(* Logix 5000 AddOnInstructionDefinition export AKD_Set_Mode; software revision 19.01 *)

TYPE AKD_Status :
STRUCT
   Profile_In_Progress : BOOL;
   Block_In_Execution : BOOL;
   On_Target_Position : BOOL;
   General_Fault : BOOL;
   Current_Direction : BOOL;
   Home_Level : BOOL;
   Reg_Level : BOOL;
   Enable : BOOL;
   Fault_Input_Fault : BOOL;
   Fwd_Limit : BOOL;
   Rev_Limit : BOOL;
   Positive_Limit : BOOL;
   Negative_Limit : BOOL;
   FE_Fault : BOOL;
   Block_Fault : BOOL;
   Load_Complete : BOOL;
END_STRUCT
END_TYPE

TYPE AKD_Control :
STRUCT
   Load_Data_Start_Profile : BOOL;
   Start_Block : BOOL;
   Incremental : BOOL;
   Direction : BOOL;
   Smooth_Stop : BOOL;
   Hard_Stop : BOOL;
   Reg_Arm : BOOL;
   Enable : BOOL;
END_STRUCT
END_TYPE

TYPE AKD_Axis :
STRUCT
   Control : AKD_Control;
   Status : AKD_Status;
   Input : AB:ETHERNET_MODULE_SINT_64Bytes:I:0;
   Output : AB:ETHERNET_MODULE_SINT_64Bytes:O:0;
   ResponseMsgType : SINT;
   CommandTimeout : INT;
   PositionFeedback : DINT;
   VelocityFeedback : DINT;
END_STRUCT
END_TYPE

ADD_ON_INSTRUCTION AKD_Get_Attribute   (* revision 2.1, ExecutePrescan, ExecuteEnableInFalse *)
VAR_OUTPUT
   DN : BOOL; {access Read Only, visible}
   ER : BOOL; {access Read Only, visible}
END_VAR
VAR_IN_OUT
   Axis : AKD_Axis; {required}
END_VAR
VAR_INPUT
   Attribute_Number : INT; {visible}
END_VAR
VAR_OUTPUT
   Attribute_Value : DINT; {access Read Only, required}
END_VAR
VAR
   Command_Timeout : TIMER := (PRE := 100);
   OS_LoadStart : BOOL;
   ErrorSource : SINT;
END_VAR

ROUTINE EnableInFalse   (* ladder *)
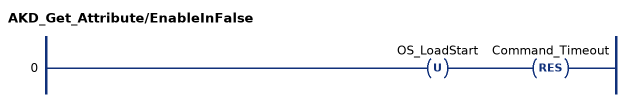
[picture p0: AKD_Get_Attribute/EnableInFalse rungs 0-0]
   0: OTU(OS_LoadStart)RES(Command_Timeout);
END_ROUTINE

ROUTINE Logic   (* ladder *)
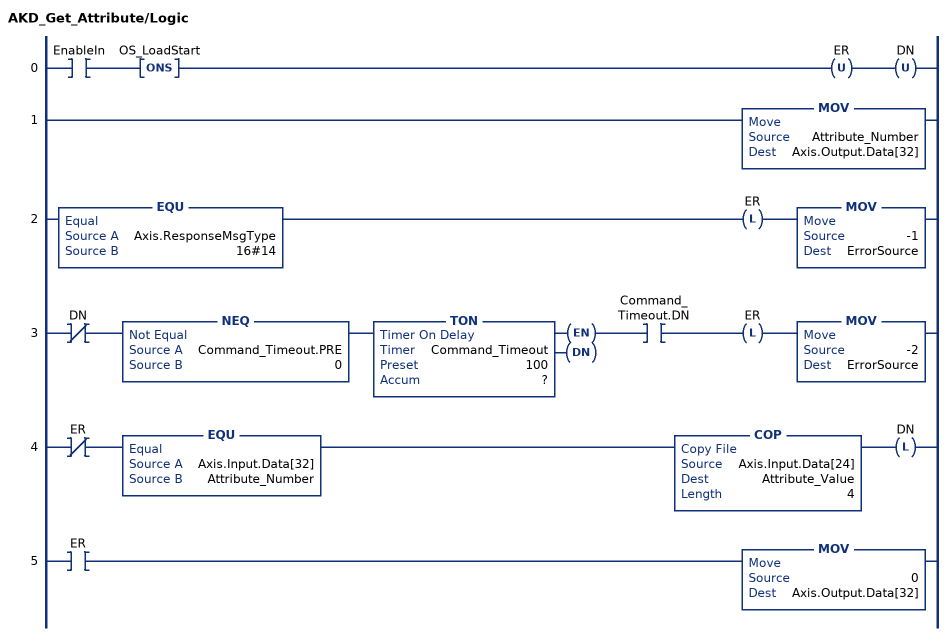
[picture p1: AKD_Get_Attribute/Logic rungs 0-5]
   0: XIC(EnableIn)ONS(OS_LoadStart)OTU(ER)OTU(DN);
   1: MOV(Attribute_Number,Axis.Output.Data[32]);
   2: EQU(Axis.ResponseMsgType,16#14)OTL(ER)MOV(-1,ErrorSource);
   3: XIO(DN)NEQ(Command_Timeout.PRE,0)TON(Command_Timeout,?,?)XIC(Command_Timeout.DN)OTL(ER)MOV(-2,ErrorSource);
   4: XIO(ER)EQU(Axis.Input.Data[32],Attribute_Number)COP(Axis.Input.Data[24],Attribute_Value,4)OTL(DN);
   5: XIC(ER)MOV(0,Axis.Output.Data[32]);
END_ROUTINE

ROUTINE Prescan   (* ladder *)
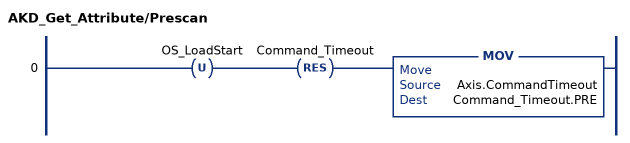
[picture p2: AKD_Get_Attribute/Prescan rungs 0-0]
   0: OTU(OS_LoadStart)RES(Command_Timeout)MOV(Axis.CommandTimeout,Command_Timeout.PRE);
END_ROUTINE
END_ADD_ON_INSTRUCTION

ADD_ON_INSTRUCTION AKD_Set_Attribute   (* revision 2.1, ExecutePrescan, ExecuteEnableInFalse *)
VAR_OUTPUT
   DN : BOOL; {access Read Only, visible}
   ER : BOOL; {access Read Only, visible}
END_VAR
VAR_IN_OUT
   Axis : AKD_Axis; {required}
END_VAR
VAR_INPUT
   Attribute_Number : INT; {visible}
   Attribute_Value : DINT; {required}
END_VAR
VAR
   Command_Timeout : TIMER := (PRE := 200);
   Command_Message_Type : SINT;
   Command_Axis_Number : SINT;
   Step : SINT;
   Command_Bytes : SINT[8];
   OS_LoadStart : BOOL;
END_VAR

ROUTINE EnableInFalse   (* ladder *)
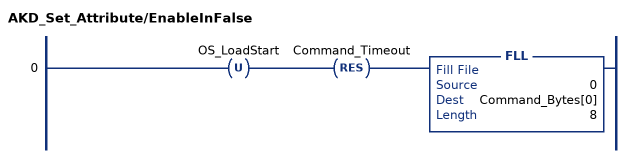
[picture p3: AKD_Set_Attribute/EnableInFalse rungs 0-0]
   0: OTU(OS_LoadStart)RES(Command_Timeout)FLL(0,Command_Bytes[0],8);
END_ROUTINE

ROUTINE Logic   (* ladder *)
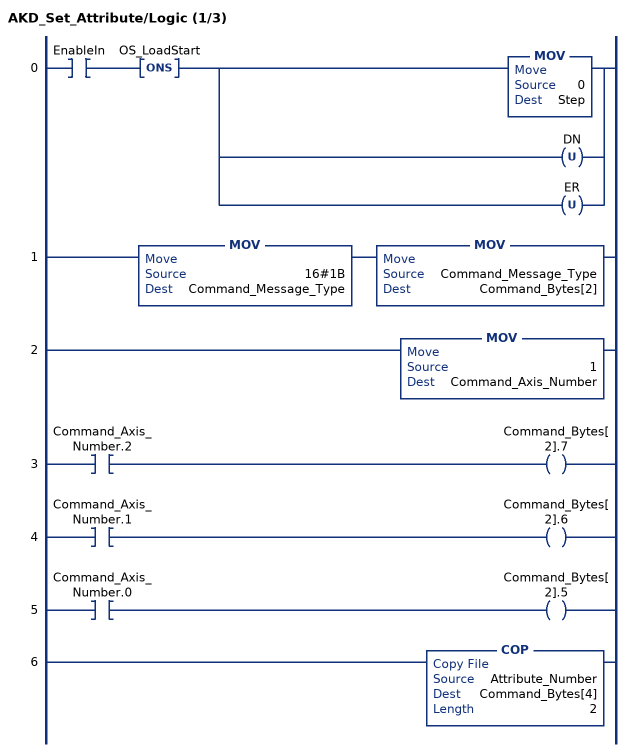
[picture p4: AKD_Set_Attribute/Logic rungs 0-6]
   0: XIC(EnableIn)ONS(OS_LoadStart)[MOV(0,Step) ,OTU(DN) ,OTU(ER) ];
   1: MOV(16#1B,Command_Message_Type)MOV(Command_Message_Type,Command_Bytes[2]);
   2: MOV(1,Command_Axis_Number);
   3: XIC(Command_Axis_Number.2)OTE(Command_Bytes[2].7);
   4: XIC(Command_Axis_Number.1)OTE(Command_Bytes[2].6);
   5: XIC(Command_Axis_Number.0)OTE(Command_Bytes[2].5);
   6: COP(Attribute_Number,Command_Bytes[4],2);
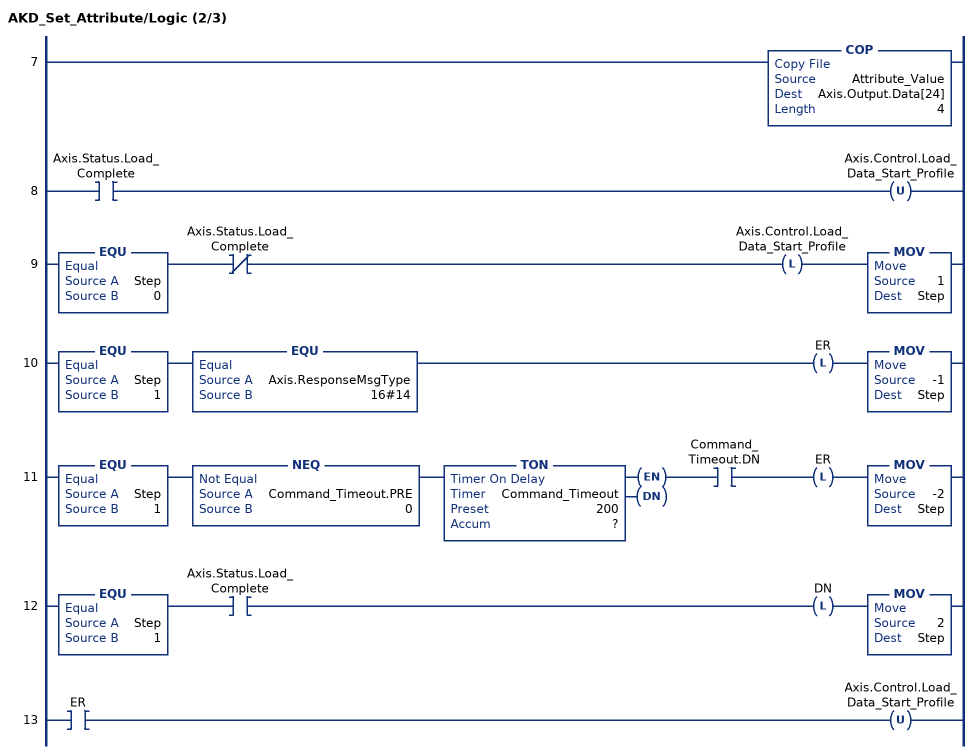
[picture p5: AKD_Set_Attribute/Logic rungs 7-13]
   7: COP(Attribute_Value,Axis.Output.Data[24],4);
   8: XIC(Axis.Status.Load_Complete)OTU(Axis.Control.Load_Data_Start_Profile);
   9: EQU(Step,0)XIO(Axis.Status.Load_Complete)OTL(Axis.Control.Load_Data_Start_Profile)MOV(1,Step);
   10: EQU(Step,1)EQU(Axis.ResponseMsgType,16#14)OTL(ER)MOV(-1,Step);
   11: EQU(Step,1)NEQ(Command_Timeout.PRE,0)TON(Command_Timeout,?,?)XIC(Command_Timeout.DN)OTL(ER)MOV(-2,Step);
   12: EQU(Step,1)XIC(Axis.Status.Load_Complete)OTL(DN)MOV(2,Step);
   13: XIC(ER)OTU(Axis.Control.Load_Data_Start_Profile);
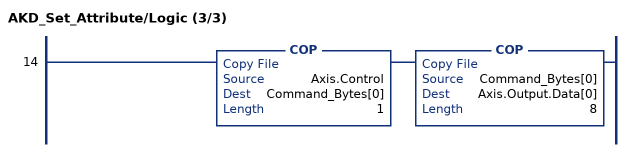
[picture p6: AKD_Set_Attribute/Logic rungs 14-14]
   14: COP(Axis.Control,Command_Bytes[0],1)COP(Command_Bytes[0],Axis.Output.Data[0],8);
END_ROUTINE

ROUTINE Prescan   (* ladder *)
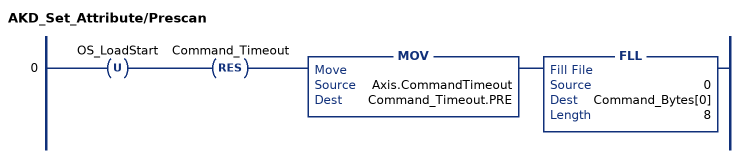
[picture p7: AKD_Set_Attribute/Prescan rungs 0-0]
   0: OTU(OS_LoadStart)RES(Command_Timeout)MOV(Axis.CommandTimeout,Command_Timeout.PRE)FLL(0,Command_Bytes[0],8);
END_ROUTINE
END_ADD_ON_INSTRUCTION

ADD_ON_INSTRUCTION AKD_Set_Mode   (* revision 4.0, ExecutePrescan, ExecuteEnableInFalse *)
// Revision note:
// Removed race with GET_MODE and SET_MODE done bit
VAR_IN_OUT
   Axis : AKD_Axis; {required}
END_VAR
VAR_INPUT
   Mode_Requested : SINT; {required}
END_VAR
VAR_OUTPUT
   DN : BOOL; {access Read Only, visible}
   ER : BOOL; {access Read Only, visible}
   Mode_Actual : SINT; {access Read Only, required}
END_VAR
VAR
   Accel_Internal : DINT;
   Step : SINT;
   ErrorSource : SINT;
   StartONS : BOOL;
   Pause_Timer : TIMER;
   Get_Mode : AKD_Get_Attribute := (Attribute_Number := 3);
   Set_Mode : AKD_Set_Attribute := (Attribute_Number := 3);
   Command_Timeout : TIMER := (PRE := 100);
END_VAR

ROUTINE EnableInFalse   (* ladder *)
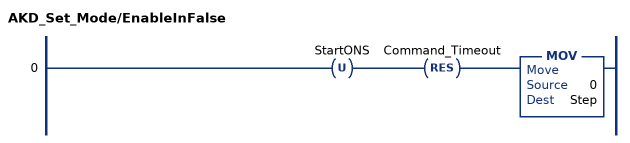
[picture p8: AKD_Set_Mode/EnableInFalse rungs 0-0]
   0: OTU(StartONS)RES(Command_Timeout)MOV(0,Step);
END_ROUTINE

ROUTINE Logic   (* ladder *)
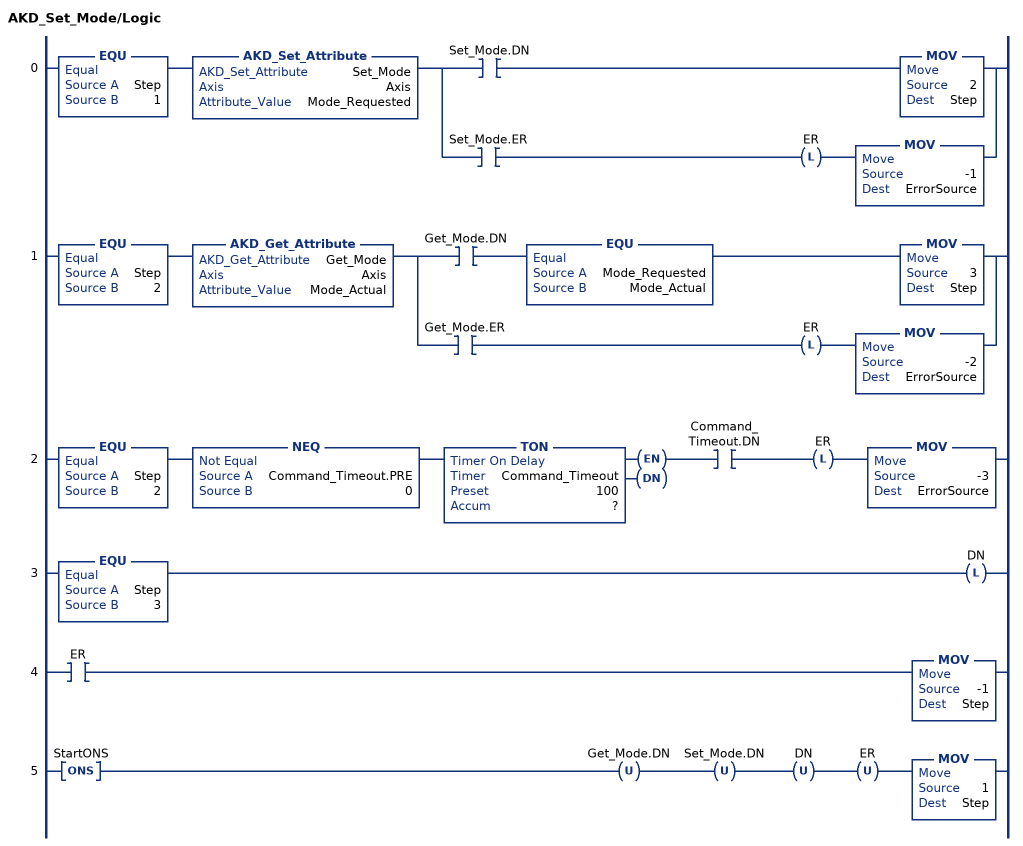
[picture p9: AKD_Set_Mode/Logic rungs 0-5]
   0: EQU(Step,1)AKD_Set_Attribute(Set_Mode,Axis,Mode_Requested)[XIC(Set_Mode.DN) MOV(2,Step) ,XIC(Set_Mode.ER) OTL(ER) MOV(-1,ErrorSource) ];
   1: EQU(Step,2)AKD_Get_Attribute(Get_Mode,Axis,Mode_Actual)[XIC(Get_Mode.DN) EQU(Mode_Requested,Mode_Actual) MOV(3,Step) ,XIC(Get_Mode.ER) OTL(ER) MOV(-2,ErrorSource) ];
   2: EQU(Step,2)NEQ(Command_Timeout.PRE,0)TON(Command_Timeout,?,?)XIC(Command_Timeout.DN)OTL(ER)MOV(-3,ErrorSource);
   3: EQU(Step,3)OTL(DN);
   4: XIC(ER)MOV(-1,Step);
   5: ONS(StartONS)OTU(Get_Mode.DN)OTU(Set_Mode.DN)OTU(DN)OTU(ER)MOV(1,Step);
END_ROUTINE

ROUTINE Prescan   (* ladder *)
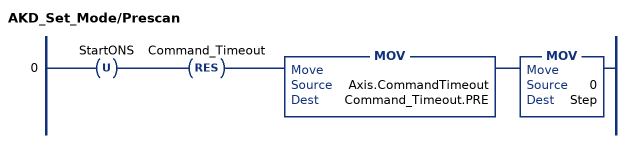
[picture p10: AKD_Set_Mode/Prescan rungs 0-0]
   0: OTU(StartONS)RES(Command_Timeout)MOV(Axis.CommandTimeout,Command_Timeout.PRE)MOV(0,Step);
END_ROUTINE
END_ADD_ON_INSTRUCTION
